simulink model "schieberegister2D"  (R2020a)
settings: Solver=VariableStepDiscrete  StartTime=0.0  StopTime=Inf  RelTol=1e-3  EnableMultiTasking=on

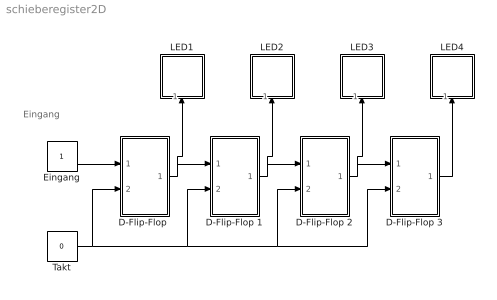
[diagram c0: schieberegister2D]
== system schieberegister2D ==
  note: Eingang
  "D-Flip-Flop " : Subsystem  mask(DFlipFlop){s0=off}
      mask prompts: s0 "Initially on"
      mask help: D Flip-Flop Block
  D-Flip-Flop 1 : Subsystem  mask(DFlipFlop){s0=off}
      mask prompts: s0 "Initially on"
      mask help: D Flip-Flop Block
  D-Flip-Flop 2 : Subsystem  mask(DFlipFlop){s0=off}
      mask prompts: s0 "Initially on"
      mask help: D Flip-Flop Block
  D-Flip-Flop 3 : Subsystem  mask(DFlipFlop){s0=off}
      mask prompts: s0 "Initially on"
      mask help: D Flip-Flop Block
  Eingang : Constant  OutDataTypeStr=double
  LED1 : Subsystem  mask(LED){on_color=[0.0, 1.0, 0.0], off_color=[0.0, 0.2, 0.0]}
      mask prompts: on_color "Color for "on" state"; off_color "Color for "off" state"
      mask help: Display of a binary signal
  LED2 : Subsystem  mask(LED){on_color=[0.0, 0.0, 1.0], off_color=[0.0, 0.5, 0.5]}
      mask prompts: on_color "Color for "on" state"; off_color "Color for "off" state"
      mask help: Display of a binary signal
  LED3 : Subsystem  mask(LED){on_color=[0.0, 1.0, 0.0], off_color=[0.0, 0.2, 0.0]}
      mask prompts: on_color "Color for "on" state"; off_color "Color for "off" state"
      mask help: Display of a binary signal
  LED4 : Subsystem  mask(LED){on_color=[0.0, 1.0, 0.0], off_color=[0.0, 0.2, 0.0]}
      mask prompts: on_color "Color for "on" state"; off_color "Color for "off" state"
      mask help: Display of a binary signal
  Takt : Constant  Value=0  OutDataTypeStr=double
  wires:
  "D-Flip-Flop "/1(Q) -> D-Flip-Flop 1/1(D), LED1/1(In)
  D-Flip-Flop 1/1(Q) -> D-Flip-Flop 2/1(D), LED2/1(In)
  D-Flip-Flop 2/1(Q) -> D-Flip-Flop 3/1(D), LED3/1(In)
  Eingang/1 -> "D-Flip-Flop "/1(D)
  Takt/1 -> "D-Flip-Flop "/2(CLK), D-Flip-Flop 1/2(CLK), D-Flip-Flop 2/2(CLK), D-Flip-Flop 3/2(CLK)
  D-Flip-Flop 3/1(Q) -> LED4/1(In)

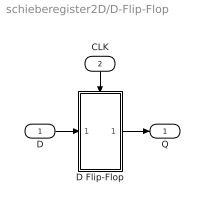
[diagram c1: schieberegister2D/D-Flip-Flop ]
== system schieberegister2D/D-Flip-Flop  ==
  D : Inport
  CLK : Inport  Port=2
  D Flip-Flop : Subsystem  TreatAsAtomicUnit=on
  Q : Outport  InitialOutput=0
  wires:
  CLK/1 -> D Flip-Flop/Trigger
  D Flip-Flop/1(Q) -> Q/1
  D/1 -> D Flip-Flop/1(D)

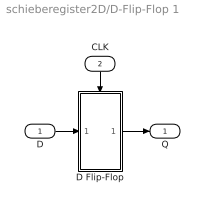
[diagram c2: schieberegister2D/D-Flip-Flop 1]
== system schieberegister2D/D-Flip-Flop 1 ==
  D : Inport
  CLK : Inport  Port=2
  D Flip-Flop : Subsystem  TreatAsAtomicUnit=on
  Q : Outport  InitialOutput=0
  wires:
  D/1 -> D Flip-Flop/1(D)
  D Flip-Flop/1(Q) -> Q/1
  CLK/1 -> D Flip-Flop/Trigger

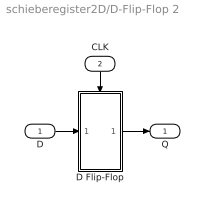
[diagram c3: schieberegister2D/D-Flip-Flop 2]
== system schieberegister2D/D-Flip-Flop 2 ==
  D : Inport
  CLK : Inport  Port=2
  D Flip-Flop : Subsystem  TreatAsAtomicUnit=on
  Q : Outport  InitialOutput=0
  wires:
  CLK/1 -> D Flip-Flop/Trigger
  D Flip-Flop/1(Q) -> Q/1
  D/1 -> D Flip-Flop/1(D)

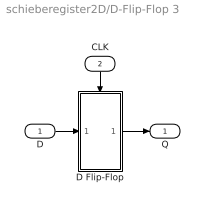
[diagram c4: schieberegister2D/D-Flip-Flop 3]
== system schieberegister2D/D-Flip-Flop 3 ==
  D : Inport
  CLK : Inport  Port=2
  D Flip-Flop : Subsystem  TreatAsAtomicUnit=on
  Q : Outport  InitialOutput=0
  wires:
  D/1 -> D Flip-Flop/1(D)
  D Flip-Flop/1(Q) -> Q/1
  CLK/1 -> D Flip-Flop/Trigger

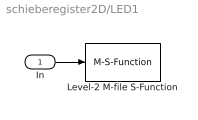
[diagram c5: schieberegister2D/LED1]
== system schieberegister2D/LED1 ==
  In : Inport
  Level-2 M-file S-Function : M-S-Function  FunctionName=sfun_setcolorD
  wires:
  In/1 -> Level-2 M-file S-Function/1

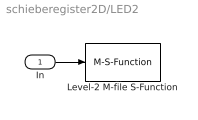
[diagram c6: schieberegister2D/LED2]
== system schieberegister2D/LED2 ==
  In : Inport
  Level-2 M-file S-Function : M-S-Function  FunctionName=sfun_setcolorD
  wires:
  In/1 -> Level-2 M-file S-Function/1

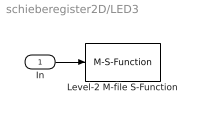
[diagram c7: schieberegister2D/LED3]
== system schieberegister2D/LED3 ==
  In : Inport
  Level-2 M-file S-Function : M-S-Function  FunctionName=sfun_setcolorD
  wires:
  In/1 -> Level-2 M-file S-Function/1

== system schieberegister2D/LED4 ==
  In : Inport
  Level-2 M-file S-Function : M-S-Function  FunctionName=sfun_setcolorD
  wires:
  In/1 -> Level-2 M-file S-Function/1

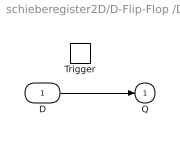
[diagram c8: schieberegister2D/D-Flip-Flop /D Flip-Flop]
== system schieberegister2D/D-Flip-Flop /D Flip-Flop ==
  D : Inport
  Trigger : TriggerPort  TriggerType=falling  VariantControl=Variant
  Q : Outport  InitialOutput=s0
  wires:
  D/1 -> Q/1

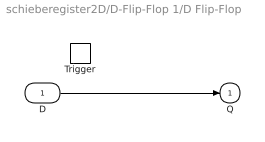
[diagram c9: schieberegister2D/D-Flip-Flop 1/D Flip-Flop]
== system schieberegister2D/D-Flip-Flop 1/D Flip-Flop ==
  D : Inport
  Trigger : TriggerPort  TriggerType=falling  VariantControl=Variant
  Q : Outport  InitialOutput=s0
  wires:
  D/1 -> Q/1

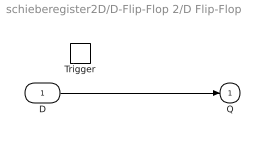
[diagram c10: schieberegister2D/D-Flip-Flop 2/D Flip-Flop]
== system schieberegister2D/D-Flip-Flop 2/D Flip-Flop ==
  D : Inport
  Trigger : TriggerPort  TriggerType=falling  VariantControl=Variant
  Q : Outport  InitialOutput=s0
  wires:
  D/1 -> Q/1

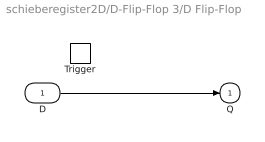
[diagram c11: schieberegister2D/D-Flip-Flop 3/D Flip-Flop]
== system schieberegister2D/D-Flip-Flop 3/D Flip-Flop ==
  D : Inport
  Trigger : TriggerPort  TriggerType=falling  VariantControl=Variant
  Q : Outport  InitialOutput=s0
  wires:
  D/1 -> Q/1
